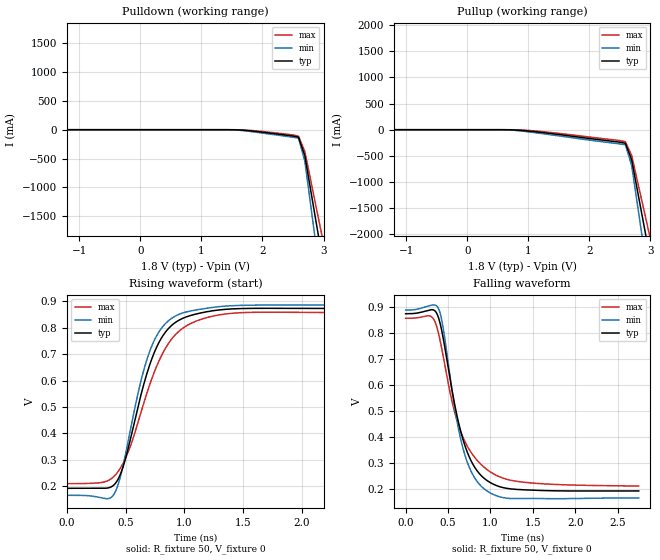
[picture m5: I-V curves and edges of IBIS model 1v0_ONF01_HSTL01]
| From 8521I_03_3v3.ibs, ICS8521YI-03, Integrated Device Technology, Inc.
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[Model]   1v0_ONF01_HSTL01
Model_type   Output_ECL
Polarity   Non-Inverting
|   typ   min   max
C_comp   2pF   1.5pF   2.5pF
Vmeas = 0.484V
Rref = 50
Cref = 0
Vref = 0V
|   typ   min   max
[Voltage range]   1.8V   1.710V   1.89V
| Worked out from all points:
|   rising waveform, R_fixture 50, V_fixture 0: 20-80 % time 262ps typ, 240ps min, 316ps max; typ from 0.192 V to 0.873 V
|   falling waveform, R_fixture 50, V_fixture 0: 20-80 % time 277ps typ, 242ps min, 338ps max; typ from 0.873 V to 0.192 V
[Pulldown]
|Voltage   I (typ)   I (min)   I (max)
-3.3V     3.779A     4.753A     3.19A
-2.887V   2.127A     2.644A     1.814A
-2.783V   1.715A     2.117A     1.471A
-2.68V    1.303A     1.591A     1.128A
-2.37V    75.44mA    45.23mA    100.8mA
-2.267V   2.573mA    1.264mA    4.791mA
2.487V    -107.3mA   -128.3mA   -88.98mA
2.693V    -451.3mA   -546.4mA   -378.1mA
2.797V    -1.096A    -1.368A    -915.7mA
2.9V      -1.74A     -2.189A    -1.454A
3.003V    -2.385A    -3.01A     -1.992A
6.6V      -26.43A    -33.51A    -22.13A
[Pullup]
|Voltage   I (typ)   I (min)   I (max)
-3.3V     3.779A     4.753A     3.19A
-2.99V    2.54A      3.171A     2.158A
-2.783V   1.715A     2.117A     1.471A
-2.37V    75.44mA    45.23mA    100.8mA
-2.267V   2.573mA    1.264mA    4.791mA
2.487V    -236.5mA   -269.8mA   -205.8mA
2.59V     -258.1mA   -288.3mA   -229.7mA
2.693V    -580.8mA   -687.5mA   -496mA
2.797V    -1.225A    -1.508A    -1.034A
2.9V      -1.869A    -2.329A    -1.572A
3.003V    -2.514A    -3.149A    -2.11A
6.6V      -25.7A     -32.68A    -21.48A
[Ramp]
|   typ   min   max
dV/dt_r   0.545/0.415n   0.587/0.383n   0.52/0.51n
dV/dt_f   0.557/0.442n   0.595/0.389n   0.523/0.563n
R_load =   50.0000
[Rising Waveform]
R_fixture = 50
V_fixture = 0
V_fixture_max = 0
V_fixture_min = 0
C_fixture = 0.0p
| Time   typ   min   max
0s        191.5mV    165mV      209mV
401.9ps   205.4mV    170.7mV    237.6mV
487.2ps   287.3mV    297.4mV    295.2mV
608.4ps   507.8mV    559mV      447.2mV
690.9ps   641.7mV    694.2mV    567mV
792.8ps   752.6mV    791.1mV    683.6mV
911.2ps   816.4mV    841.5mV    768.2mV
1.087ns   850.8mV    866.7mV    823mV
1.371ns   870.7mV    882.9mV    853.5mV
2.747ns   872.9mV    886.7mV    856.5mV
[Falling Waveform]
R_fixture = 50
V_fixture = 0
V_fixture_max = 0
V_fixture_min = 0
C_fixture = 0.0p
| Time   typ   min   max
0s        872.8mV    886.9mV    855.3mV
294.5ps   887.9mV    904.8mV    863.3mV
388.1ps   857mV      892mV      796.8mV
443.2ps   778.5mV    816.8mV    708.7mV
547.8ps   577.3mV    574.6mV    534.3mV
666.2ps   400.4mV    367.7mV    405.4mV
779ps     302.6mV    262.1mV    336.1mV
927.7ps   239.6mV    199.1mV    282.1mV
1.371ns   196.4mV    162.7mV    226.1mV
2.747ns   191.7mV    164.9mV    210.8mV
